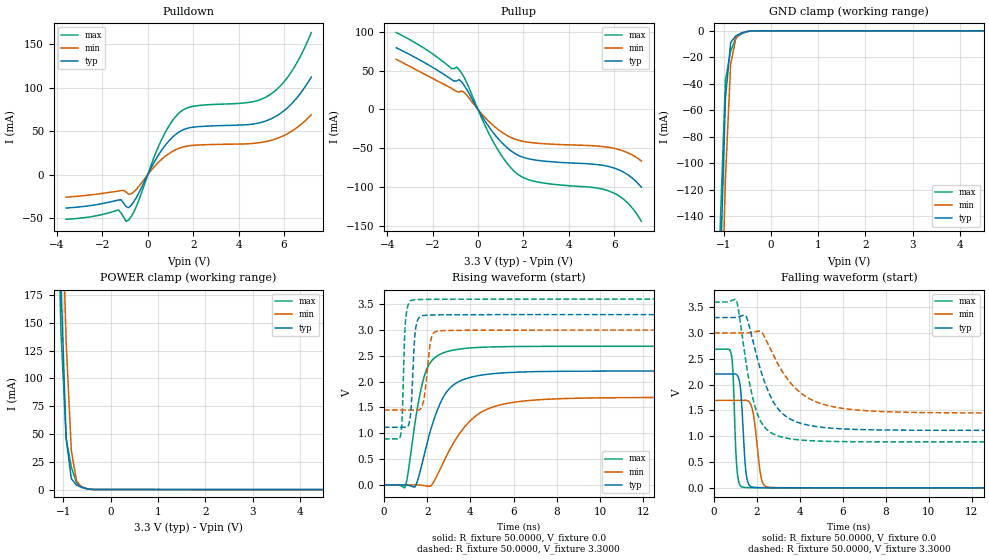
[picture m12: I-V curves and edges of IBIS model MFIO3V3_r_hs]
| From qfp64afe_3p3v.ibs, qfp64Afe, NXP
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[Model] MFIO3V3_r_hs
|   Model MFIO3V3_r_hs
| This model was characterised for following simulation conditions:
| External (pad) voltage:
|   - Typ: 3.3V,   - Min: 3.0V,   - Max: 3.6V
| Library cells for typ/min/max conditions are connected as defined below:
|  IO - External Pad
|  A - Core Input
|  EN - Output Buffer Enable
|  BOOST - vdde
|  EHS - vdd
|  ENZI - vdd
|  EPD - vdd
|  EPUN - gnd
|  ZI - NC
|  ZIF - NC
|  gnd - gnd
|  gnde - gnde
|  vdd - vdd
|  vdde - vdde
| All other pins connected to ground
Model_type I/O
Polarity   Non-Inverting
Enable   Active-Low
Vinl =   0.9900V
Vinh =   2.3100V
Vmeas =  1.6500V
Cref =   0.0F
Rref =   100.0000
Vref =   0.0V
C_comp   1.5343pF   1.4580pF   1.6019pF
|C_comp_pullup   0.7283pF   0.7532pF   0.6914pF
|C_comp_pulldown   0.5932pF   0.6316pF   0.5575pF
[Model Spec]
| variable   typ   min   max
Vinh   0.9900V   0.9000V   1.0800V
Vinl   2.3100V   2.1000V   2.5200V
Vmeas   1.6500V   1.5000V   1.8000V
[Temperature Range]   25.0000   0.1250k   -40.0000
[Voltage Range]   3.3000V   3.0000V   3.6000V
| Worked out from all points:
|   slope of the pulldown table from 0 to 0.495 V, typ, clamps not added: 21 ohm
|   slope of the pullup table from 0 to 0.495 V, typ, clamps not added: 21.7 ohm
|   GND clamp passes 1 mA (typ) near -0.56 V on its own axis
|   POWER clamp passes 1 mA (typ) near -0.53 V on its own axis
|   rising waveform, R_fixture 50.0000, V_fixture 0.0: 20-80 % time 1.06ns typ, 1.67ns min, 677ps max; typ from 0 V to 2.21 V
|   rising waveform, R_fixture 50.0000, V_fixture 3.3000: 20-80 % time 158ps typ, 234ps min, 125ps max; typ from 1.11 V to 3.3 V
|   falling waveform, R_fixture 50.0000, V_fixture 0.0: 20-80 % time 188ps typ, 278ps min, 145ps max; typ from 2.21 V to 0 V
|   falling waveform, R_fixture 50.0000, V_fixture 3.3000: 20-80 % time 1.14ns typ, 1.68ns min, 747ps max; typ from 3.3 V to 1.11 V
[Pulldown]
|Voltage   I(typ)   I(min)   I(max)
-3.6V     -38.54mA   -26.03mA   -51.47mA
-1.29V    -29.27mA   -18.96mA   -40.78mA
-960mV    -36.81mA   -20.01mA   -53.83mA
-850mV    -38.18mA   -22.68mA   -52.4mA
-520mV    -27.12mA   -17.5mA    -37.74mA
580mV     26.98mA    16.83mA    38.78mA
1.35V     48.62mA    30.01mA    70.27mA
2.01V     54.62mA    33.69mA    78.71mA
4.43V     57.57mA    35.54mA    83.11mA
5.31V     62.85mA    38.64mA    90.87mA
6.3V      80.67mA    49.35mA    117.4mA
7.2V      112.3mA    68.85mA    163.6mA
[Pullup]
|Voltage   I(typ)   I(min)   I(max)
-3.6V     79.43mA    64.59mA    99.03mA
-1.05V    36.46mA    25.05mA    52.51mA
-830mV    38.41mA    22.29mA    50.98mA
-610mV    31.13mA    22.16mA    41.54mA
270mV     -13.03mA   -9.075mA   -18mA
710mV     -31.29mA   -21.6mA    -43.53mA
1.26V     -48.73mA   -33.16mA   -68.54mA
1.7V      -58.01mA   -38.97mA   -82.27mA
2.58V     -65.44mA   -43.49mA   -93.28mA
5.88V     -74.5mA    -49.46mA   -106.4mA
6.65V     -85.19mA   -56.54mA   -122.1mA
7.2V      -100.2mA   -66.51mA   -144.2mA
[GND_clamp]
|Voltage   I(typ)   I(min)   I(max)
-3.6V     -4.776A    -4.755A    -4.803A
-1.07V    -185.2mA   -255.8mA   -147.9mA
-960mV    -51.26mA   -111.8mA   -37.36mA
-850mV    -8.879mA   -25.45mA   -15.19mA
-740mV    -3.782mA   -5.531mA   -5.645mA
-630mV    -1.803mA   -1.784mA   -2.444mA
-520mV    -592.1uA   -582.6uA   -781uA
-300mV    -8.619uA   -12.3uA    -9.227uA
7.2V      0A         0A         0A
[POWER_clamp]
|Voltage   I(typ)   I(min)   I(max)
-3.6V     5.691A     5.665A     5.731A
-1.16V    387.4mA    485.6mA    339.3mA
-1.05V    187.9mA    295.9mA    142.8mA
-940mV    46.42mA    133mA      46.27mA
-830mV    9.779mA    35.03mA    20.21mA
-720mV    4.043mA    7.776mA    6.047mA
-610mV    1.916mA    2.078mA    2.613mA
-500mV    646.2uA    680.9uA    832.2uA
-280mV    73uA       65.71uA    91.35uA
7.2V      0A         0A         0A
[Ramp]
| variable   typ   min   max
dV/dt_r  1.3230/1.0597n   1.0165/1.6685n   1.6111/0.6773n
dV/dt_f  1.3109/1.1397n   0.9294/1.6808n   1.6255/0.7471n
R_load = 50.0000
[Rising Waveform]
R_fixture= 50.0000
V_fixture= 0.0
V_fixture_min= 0.0
V_fixture_max= 0.0
|time   V(typ)   V(min)   V(max)
0s        3.835nV    108.6nV    40.83nV
985.9ps   46.31uV    -26.41uV   -34.32mV
1.468ns   -16.04mV   257.4uV    1.29V
1.791ns   459.1mV    -10.13mV   1.993V
2.134ns   1.024V     -25.87mV   2.365V
2.894ns   1.798V     559.6mV    2.579V
4.214ns   2.104V     1.323V     2.659V
5.961ns   2.18V      1.597V     2.68V
10.33ns   2.204V     1.688V     2.685V
100ns     2.205V     1.694V     2.685V
[Rising Waveform]
R_fixture= 50.0000
V_fixture= 3.3000
V_fixture_min= 3.0000
V_fixture_max= 3.6000
|time   V(typ)   V(min)   V(max)
0s        1.114V     1.45V      889.8mV
777.6ps   1.114V     1.45V      976.5mV
848.6ps   1.114V     1.45V      1.372V
974.8ps   1.113V     1.45V      3.034V
1.152ns   1.176V     1.45V      3.525V
1.453ns   2.988V     1.448V     3.588V
1.828ns   3.282V     1.619V     3.594V
2.212ns   3.292V     2.876V     3.596V
2.77ns    3.295V     2.989V     3.597V
100ns     3.299V     2.999V     3.599V
[Falling Waveform]
R_fixture= 50.0000
V_fixture= 0.0
V_fixture_min= 0.0
V_fixture_max= 0.0
|time   V(typ)   V(min)   V(max)
0s        2.205V     1.694V     2.685V
791.4ps   2.205V     1.694V     2.607V
876.2ps   2.206V     1.694V     2.273V
1.077ns   2.183V     1.694V     315mV
1.245ns   1.862V     1.694V     29.43mV
1.452ns   438.9mV    1.698V     6.832mV
1.799ns   13.32mV    1.495V     2.986mV
2.241ns   3.742mV    122.6mV    1.708mV
2.707ns   2.12mV     7.124mV    1.062mV
100ns     10.27nV    120nV      44.8nV
[Falling Waveform]
R_fixture= 50.0000
V_fixture= 3.3000
V_fixture_min= 3.0000
V_fixture_max= 3.6000
|time   V(typ)   V(min)   V(max)
0s        3.299V     2.999V     3.599V
1.048ns   3.307V     2.999V     3.627V
1.514ns   3.305V     3.001V     2.358V
1.868ns   2.751V     3.02V      1.631V
2.246ns   2.18V      3.002V     1.237V
3.062ns   1.491V     2.334V     994.6mV
4.341ns   1.218V     1.75V      917mV
6.38ns    1.135V     1.519V     894mV
10.45ns   1.115V     1.456V     889.9mV
100ns     1.114V     1.45V      889.8mV
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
